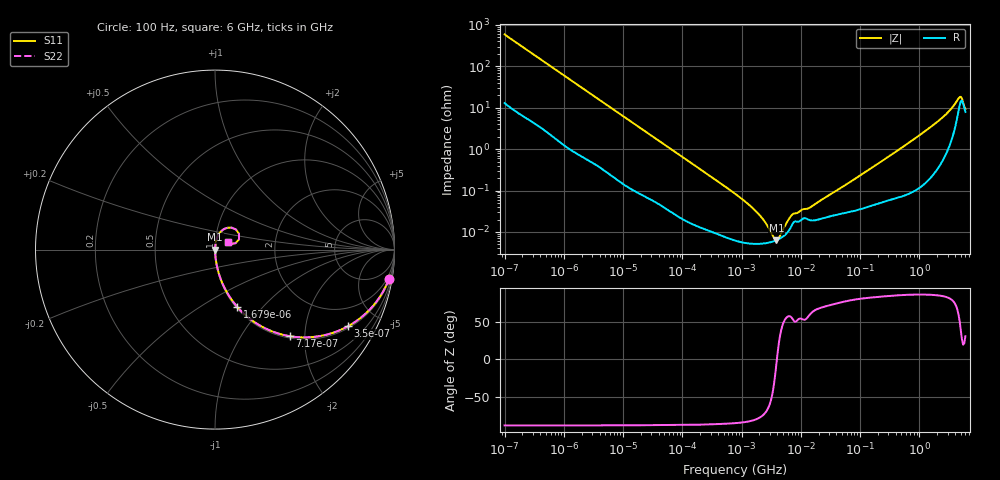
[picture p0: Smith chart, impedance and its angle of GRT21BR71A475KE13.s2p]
!Murata Part Number: GRT21BR71A475KE13
!These Parameters are Measured in Series Mode Connection
!Data Generated on Jun 19, 2026
!  o--ll--o
!Port1  Port2
!  o------o
!Operation Temp=25[degC], DC Bias Voltage=0[V]
!Freq. Start=100[Hz] Stop=6[GHz] 401[Steps]
# Hz S RI R 50
!Freq.(Hz) S11(Real) S11(Imag) S21(Real) S21(Imag) S12(Real) S12(Imag) S22(Real) S22(Imag)
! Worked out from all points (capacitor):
!   401 points, 100 Hz to 6 GHz, reference 50 ohm
!   read as one part in series: C = 2.69 uF near 109 Hz
!   lowest |Z| = 6.34 mohm at 3.882 MHz (marker M1)
!   series resonance near 3.949 MHz, so ESL is about 600 pH
!   S11 on the Smith chart (normalised r, x): 100 Hz: 1, -12; 350 Hz: 1.08, -3.42; 717 Hz: 1.04, -1.69; 1.679 kHz: 1.02, -0.73; 6 GHz: 1.16, +0.10
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100  0.9687 -0.1636  0.0313 0.1636  0.0313 0.1636  0.9687 -0.1636
196  0.897 -0.2934  0.103 0.2934  0.103 0.2934  0.897 -0.2934
350  0.7404 -0.4273  0.2596 0.4273  0.2596 0.4273  0.7404 -0.4273
717  0.418 -0.4827  0.582 0.4827  0.582 0.4827  0.418 -0.4827
1122  0.2319 -0.4119  0.7681 0.4119  0.7681 0.4119  0.2319 -0.4119
1679  0.1222 -0.3171  0.8778 0.3171  0.8778 0.3171  0.1222 -0.3171
2008  0.0901 -0.2757  0.9099 0.2757  0.9099 0.2757  0.0901 -0.2757
7036  0.00982 -0.0877  0.9902 0.0877  0.9902 0.0877  0.00982 -0.0877
40335  0.000718 -0.0159  0.9993 0.0159  0.9993 0.0159  0.000718 -0.0159
774597  6.27e-05 -0.000839  0.9999 0.000839  0.9999 0.000839  6.27e-05 -0.000839
1813585  5.15e-05 -0.000297  0.9999 0.000297  0.9999 0.000297  5.15e-05 -0.000297
3103719  5.66e-05 -8.44e-05  0.9999 8.44e-05  0.9999 8.44e-05  5.66e-05 -8.44e-05
3882480  6.31e-05 -5.9e-06  0.9999 5.9e-06  0.9999 5.9e-06  6.31e-05 -5.9e-06
4856642  7.49e-05 7.36e-05  0.9999 -7.36e-05  0.9999 -7.36e-05  7.49e-05 7.36e-05
7266822  0.000157 0.000218  0.9998 -0.000218  0.9998 -0.000218  0.000157 0.000218
1.555665e7  0.000189 0.000376  0.9998 -0.000376  0.9998 -0.000376  0.000189 0.000376
3.124326e8  0.000632 0.00677  0.9994 -0.00677  0.9994 -0.00677  0.000632 0.00677
2.048624e9  0.00551 0.0461  0.9945 -0.0461  0.9945 -0.0461  0.00551 0.0461
3.505958e9  0.025 0.0912  0.975 -0.0912  0.975 -0.0912  0.025 0.0912
4.586474e9  0.0928 0.1222  0.9072 -0.1222  0.9072 -0.1222  0.0928 0.1222
5.016141e9  0.1338 0.0883  0.8662 -0.0883  0.8662 -0.0883  0.1338 0.0883
6e9  0.0751 0.0408  0.9249 -0.0408  0.9249 -0.0408  0.0751 0.0408
